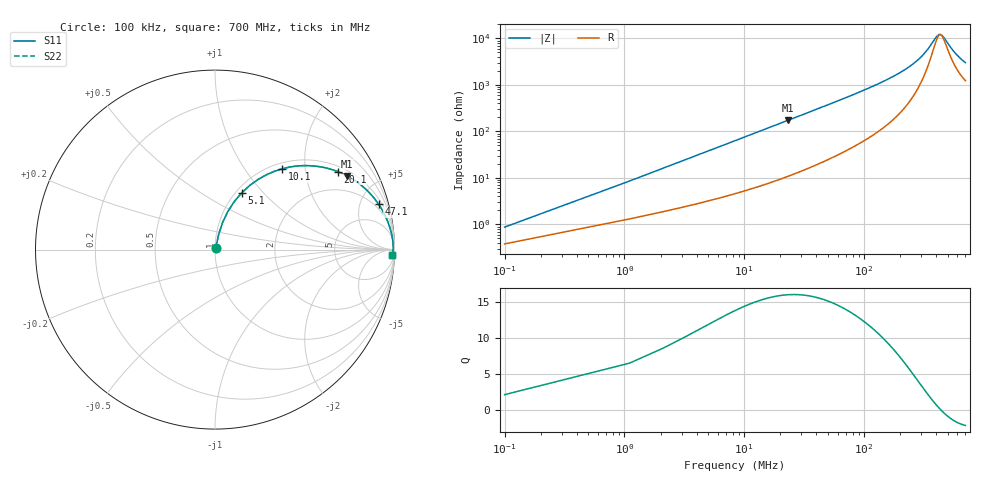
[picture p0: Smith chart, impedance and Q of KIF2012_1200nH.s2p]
!version-2
!date-12.2020
!Series
# MHz S RI R 50
!Freq ReS11 ImS11 ReS21 ImS21 ReS12 ImS12 ReS22 ImS22
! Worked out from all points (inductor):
!   701 points, 100 kHz to 700 MHz, reference 50 ohm
!   read as one part in series: L = 1.21 uH near 3.1 MHz
!   highest Q = 15.9 at 23.1 MHz (marker M1), where L = 1.19 uH
!   self-resonance near 433.8 MHz
!   S11 on the Smith chart (normalised r, x): 100 kHz: 1.01, +0.02; 5.1 MHz: 1.06, +0.77; 10.1 MHz: 1.11, +1.52; 20.1 MHz: 1.19, +3.00; 47.1 MHz: 1.46, +7.04; 700 MHz: 26, -55
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0.1  0.00386 0.00783  0.9961 -0.00783  0.9961 -0.00783  0.00386 0.00783
2.1  0.0422 0.1509  0.9578 -0.1509  0.9578 -0.1509  0.0422 0.1509
4.1  0.109 0.2697  0.891 -0.2697  0.891 -0.2697  0.109 0.2697
5.1  0.1503 0.3178  0.8497 -0.3178  0.8497 -0.3178  0.1503 0.3178
7.1  0.2404 0.3911  0.7596 -0.3911  0.7596 -0.3911  0.2404 0.3911
10.1  0.3752 0.4507  0.6248 -0.4507  0.6248 -0.4507  0.3752 0.4507
15.1  0.5585 0.4652  0.4415 -0.4652  0.4415 -0.4652  0.5585 0.4652
20.1  0.6831 0.4348  0.3169 -0.4348  0.3169 -0.4348  0.6831 0.4348
23.1  0.7363 0.4104  0.2637 -0.4104  0.2637 -0.4104  0.7363 0.4104
33.1  0.8444 0.3323  0.1556 -0.3323  0.1556 -0.3323  0.8444 0.3323
47.1  0.9114 0.2532  0.0886 -0.2532  0.0886 -0.2532  0.9114 0.2532
77.1  0.9604 0.1615  0.0396 -0.1615  0.0396 -0.1615  0.9604 0.1615
117.1  0.9794 0.1045  0.0206 -0.1045  0.0206 -0.1045  0.9794 0.1045
234.1  0.9913 0.0406  0.00874 -0.0406  0.00874 -0.0406  0.9913 0.0406
350.1  0.9925 0.0133  0.0075 -0.0133  0.0075 -0.0133  0.9925 0.0133
394.1  0.9922 0.00591  0.00776 -0.00591  0.00776 -0.00591  0.9922 0.00591
417.1  0.992 0.00241  0.00799 -0.00241  0.00799 -0.00241  0.992 0.00241
439.1  0.9917 -0.00075  0.00827 0.00075  0.00827 0.00075  0.9917 -0.00075
467.1  0.9913 -0.00453  0.00869 0.00453  0.00869 0.00453  0.9913 -0.00453
527.1  0.9902 -0.0119  0.00982 0.0119  0.00982 0.0119  0.9902 -0.0119
584.1  0.9889 -0.0182  0.0111 0.0182  0.0111 0.0182  0.9889 -0.0182
700  0.9856 -0.0294  0.0144 0.0294  0.0144 0.0294  0.9856 -0.0294
